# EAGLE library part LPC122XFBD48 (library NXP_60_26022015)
NXP ARM M0 32 bit Microcontroller AAL Eindhoven MV+ MK
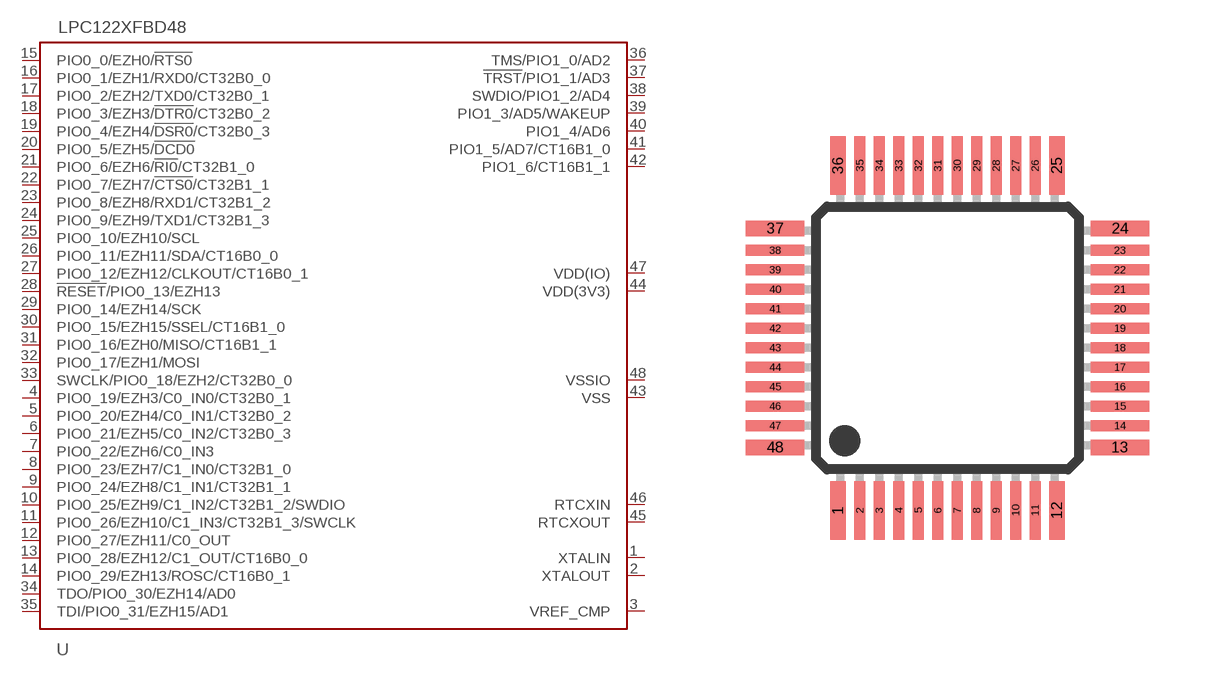
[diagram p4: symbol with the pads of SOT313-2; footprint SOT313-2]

Designator prefix U

## LPC122XFBD48  [SOT313-2]
1  XTALIN
2  XTALOUT
3  VREF_CMP
4  PIO0_19/EZH3/C0_IN0/CT32B0_1
5  PIO0_20/EZH4/C0_IN1/CT32B0_2
6  PIO0_21/EZH5/C0_IN2/CT32B0_3
7  PIO0_22/EZH6/C0_IN3
8  PIO0_23/EZH7/C1_IN0/CT32B1_0
9  PIO0_24/EZH8/C1_IN1/CT32B1_1
10  PIO0_25/EZH9/C1_IN2/CT32B1_2/SWDIO
11  PIO0_26/EZH10/C1_IN3/CT32B1_3/SWCLK
12  PIO0_27/EZH11/C0_OUT
13  PIO0_28/EZH12/C1_OUT/CT16B0_0
14  PIO0_29/EZH13/ROSC/CT16B0_1
15  PIO0_0/EZH0/!RTS0!
16  PIO0_1/EZH1/RXD0/CT32B0_0
17  PIO0_2/EZH2/TXD0/CT32B0_1
18  PIO0_3/EZH3/!DTR0!/CT32B0_2
19  PIO0_4/EZH4/!DSR0!/CT32B0_3
20  PIO0_5/EZH5/!DCD0!
21  PIO0_6/EZH6/!RI0!/CT32B1_0
22  PIO0_7/EZH7/!CTS0!/CT32B1_1
23  PIO0_8/EZH8/RXD1/CT32B1_2
24  PIO0_9/EZH9/TXD1/CT32B1_3
25  PIO0_10/EZH10/SCL
26  PIO0_11/EZH11/SDA/CT16B0_0
27  PIO0_12/EZH12/CLKOUT/CT16B0_1
28  !RESET!/PIO0_13/EZH13
29  PIO0_14/EZH14/SCK
30  PIO0_15/EZH15/SSEL/CT16B1_0
31  PIO0_16/EZH0/MISO/CT16B1_1
32  PIO0_17/EZH1/MOSI
33  SWCLK/PIO0_18/EZH2/CT32B0_0
34  TDO/PIO0_30/EZH14/AD0
35  TDI/PIO0_31/EZH15/AD1
36  TMS/PIO1_0/AD2
37  !TRST!/PIO1_1/AD3
38  SWDIO/PIO1_2/AD4
39  PIO1_3/AD5/WAKEUP
40  PIO1_4/AD6
41  PIO1_5/AD7/CT16B1_0
42  PIO1_6/CT16B1_1
43  VSS  pwr
44  VDD(3V3)  pwr
45  RTCXOUT
46  RTCXIN
47  VDD(IO)  pwr
48  VSSIO  pwr

## Footprint SOT313-2 (pad centres in mm)
SOT313-2 LQFP48: plastic low profile quad flat package; 48 leads; body 7 x 7 x 1.4 mm JEDEC: MS-026 IEC: 136E05 Footprint according to NXP SOT313-2 specification, however the cornerpins are 0.4mm in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
smd 0.4 x 1.5: 1 -2.81,-4.425; 12 2.81,-4.425; 25 2.81,4.425; 36 -2.81,4.425
smd 0.28 x 1.5: 2 -2.25,-4.425; 3 -1.75,-4.425; 4 -1.25,-4.425; 5 -0.75,-4.425; 6 -0.25,-4.425; 7 0.25,-4.425; 8 0.75,-4.425; 9 1.25,-4.425; 10 1.75,-4.425; 11 2.25,-4.425; 26 2.25,4.425; 27 1.75,4.425; 28 1.25,4.425; 29 0.75,4.425; 30 0.25,4.425; 31 -0.25,4.425; 32 -0.75,4.425; 33 -1.25,4.425; 34 -1.75,4.425; 35 -2.25,4.425
smd 1.5 x 0.4: 13 4.425,-2.81; 24 4.425,2.81; 37 -4.425,2.81; 48 -4.425,-2.81
smd 1.5 x 0.28: 14 4.425,-2.25; 15 4.425,-1.75; 16 4.425,-1.25; 17 4.425,-0.75; 18 4.425,-0.25; 19 4.425,0.25; 20 4.425,0.75; 21 4.425,1.25; 22 4.425,1.75; 23 4.425,2.25; 38 -4.425,2.25; 39 -4.425,1.75; 40 -4.425,1.25; 41 -4.425,0.75; 42 -4.425,0.25; 43 -4.425,-0.25; 44 -4.425,-0.75; 45 -4.425,-1.25; 46 -4.425,-1.75; 47 -4.425,-2.25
